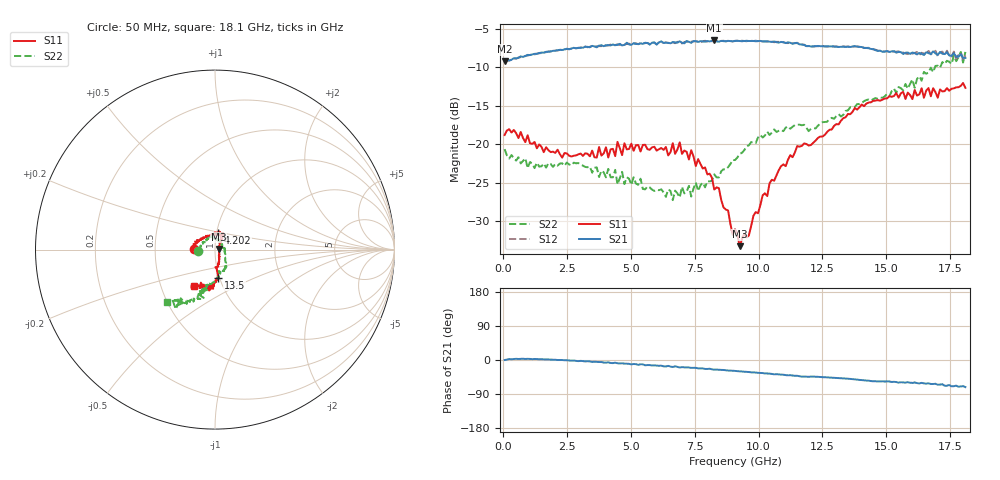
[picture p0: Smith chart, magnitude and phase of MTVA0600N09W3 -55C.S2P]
! Network Analyzer HP8720D.06.14 Serial No. US36140669
! 10 May 2005  14:46:33
! Frequency  S11  S21  S12  S22
# HZ  S  DB R 50
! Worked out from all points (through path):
!   201 points, 50 MHz to 18.1 GHz, reference 50 ohm
!   highest |S21| = -6.53 dB at 8.263 GHz (marker M1); lowest = -9.3 dB at 50 MHz (marker M2)
!   group delay of S21, straight-line fit = 12.1 ps
!   lowest |S11| = -33.3 dB at 9.255 GHz (marker M3), VSWR 1.04, Z = 52.2 + j0.302 ohm
!   |S11| at or under -10 dB: start of sweep to end of sweep
!   |S22| runs from -27.3 to -8.0 dB; largest |S21 - S12| = 0.019
!   S11 on the Smith chart (normalised r, x): 50 MHz: 0.79, +0.01; 4.202 GHz: 1.02, +0.19; 13.5 GHz: 0.99, -0.32; 18.1 GHz: 0.74, -0.31
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5e7  -18.82 177.4  -9.25 -0.0  -9.29 -0.3  -20.66 -176.8
9.525e8  -18.85 152.4  -8.40 3.1  -8.49 2.9  -23.13 144.5
1.58425e9  -21.05 136.0  -8.12 1.7  -8.09 1.5  -22.52 126.0
3.1185e9  -21.54 100.8  -7.47 -2.9  -7.48 -3.4  -22.80 107.8
4.2015e9  -20.70 79.0  -7.18 -7.9  -7.06 -7.7  -24.31 93.6
6.09675e9  -20.66 67.5  -6.78 -15.2  -6.75 -15.5  -26.00 48.9
6.63825e9  -19.89 66.5  -6.75 -18.3  -6.76 -17.9  -27.29 28.0
6.7285e9  -21.27 70.5  -6.77 -16.7  -6.89 -17.4  -26.05 25.0
6.909e9  -19.78 63.8  -6.64 -19.7  -6.71 -19.3  -26.93 16.8
7.27e9  -22.00 57.9  -6.70 -19.6  -6.79 -20.8  -25.43 10.1
7.36025e9  -20.80 55.5  -6.84 -20.7  -6.69 -20.8  -26.83 12.7
8.26275e9  -25.91 55.1  -6.53 -25.5  -6.68 -25.6  -23.94 -23.8
8.44325e9  -25.73 54.6  -6.69 -25.8  -6.59 -25.6  -24.33 -28.1
8.98475e9  -31.78 26.8  -6.65 -28.2  -6.66 -28.4  -22.07 -42.2
9.075e9  -31.07 18.8  -6.59 -29.0  -6.58 -29.4  -22.08 -44.0
9.2555e9  -33.27 7.6  -6.60 -30.0  -6.64 -30.4  -21.27 -47.3
1.088e10  -22.86 -71.6  -6.72 -38.5  -6.76 -39.2  -18.16 -64.2
1.21435e10  -19.82 -84.9  -7.32 -43.5  -7.29 -44.2  -17.95 -77.1
1.349725e10  -16.09 -83.5  -7.34 -49.4  -7.33 -49.8  -15.62 -85.2
1.512175e10  -13.78 -93.6  -8.02 -56.7  -8.01 -57.5  -13.79 -102.0
1.656575e10  -13.05 -107.5  -8.07 -62.4  -8.34 -62.5  -10.85 -106.6
1.81e10  -12.70 -120.1  -8.81 -71.5  -8.50 -72.8  -8.02 -132.3
